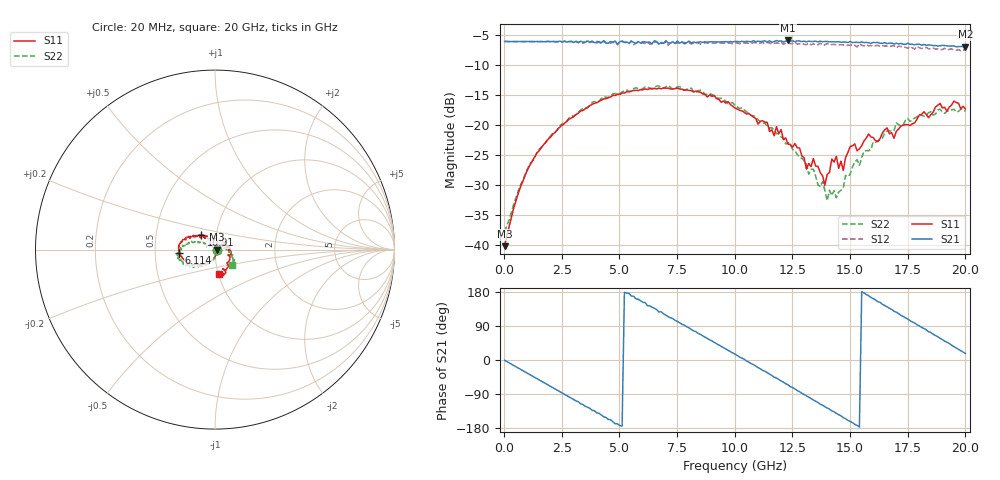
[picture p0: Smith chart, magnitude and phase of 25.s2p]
!Agilent Technologies,N5230A,US43500223,A.07.50.48
!Agilent N5230A: A.07.50.48
!Date: Wednesday, October 07, 2015 12:05:37
!Correction: S11(Full 2 Port(1,2))
!S21(Full 2 Port(1,2))
!S12(Full 2 Port(1,2))
!S22(Full 2 Port(1,2))
!S2P File: Measurements: S11, S21, S12, S22:
# Hz S  RI  R 50
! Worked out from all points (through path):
!   201 points, 20 MHz to 20 GHz, reference 50 ohm
!   highest |S21| = -5.91 dB at 12.31 GHz (marker M1); lowest = -7.0 dB at 20 GHz (marker M2)
!   group delay of S21, straight-line fit = 97.4 ps
!   lowest |S11| = -40.2 dB at 20 MHz (marker M3), VSWR 1.02, Z = 51 - j0.0154 ohm
!   |S11| at or under -10 dB: start of sweep to end of sweep
!   |S22| runs from -37.8 to -13.4 dB; largest |S21 - S12| = 0.056
!   S11 on the Smith chart (normalised r, x): 20 MHz: 1.02, -0.00; 6.114 GHz: 0.67, -0.03; 10.91 GHz: 0.84, +0.14; 20 GHz: 1.01, -0.28
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2e7  0.00981 -0.000151  0.4972 -0.00634  0.4965 -0.00734  0.0129 -0.00112
6.194e8  0.00632 -0.0266  0.4615 -0.1812  0.4601 -0.1829  0.00927 -0.0271
1.4186e9  -0.0137 -0.0568  0.326 -0.3746  0.3217 -0.3763  -0.0116 -0.0579
2.6174e9  -0.0629 -0.0821  -0.00392 -0.4998  -0.0122 -0.5011  -0.0555 -0.0869
3.4166e9  -0.103 -0.0832  -0.2276 -0.4358  -0.2377 -0.4169  -0.0965 -0.0981
4.8152e9  -0.1662 -0.0593  -0.4906 -0.1042  -0.4909 -0.0935  -0.1603 -0.0881
6.1139e9  -0.1992 -0.0185  -0.4338 0.2341  -0.4117 0.2409  -0.2007 -0.0541
6.7133e9  -0.2029 0.00205  -0.283 0.3785  -0.2688 0.3855  -0.2064 -0.0479
8.012e9  -0.1899 0.0406  0.0446 0.4981  0.0683 0.4819  -0.2032 -0.00274
1.001e10  -0.1189 0.0715  0.4798 0.1304  0.474 0.1028  -0.1404 0.0372
1.09091e10  -0.0783 0.0822  0.474 -0.1365  0.4534 -0.1716  -0.1091 0.0412
1.23077e10  -0.0348 0.0601  0.2105 -0.4605  0.1657 -0.4573  -0.0613 0.0364
1.28072e10  -0.0247 0.0596  0.0567 -0.4978  0.0229 -0.4746  -0.0439 0.0316
1.31069e10  -0.0103 0.0418  -0.0405 -0.4905  -0.0639 -0.4631  -0.034 0.034
1.34066e10  -0.006 0.0524  -0.1335 -0.4782  -0.1559 -0.4483  -0.0287 0.0321
1.39061e10  0.01 0.0299  -0.2726 -0.415  -0.2741 -0.3758  -0.00695 0.0278
1.44056e10  0.0464 0.0293  -0.3824 -0.3094  -0.3828 -0.2655  0.00935 0.023
1.47053e10  0.0359 0.0219  -0.4341 -0.2293  -0.423 -0.1915  0.022 0.0205
1.5005e10  0.0622 0.0234  -0.4729 -0.1518  -0.444 -0.1209  0.0363 0.0141
1.67033e10  0.0781 -0.0328  -0.3485 0.3311  -0.3097 0.324  0.0883 -0.017
1.82018e10  0.0615 -0.1137  0.0568 0.4652  0.0768 0.434  0.0977 -0.0671
2e10  0.024 -0.134  0.4282 0.1328  0.4154 0.0863  0.0974 -0.0861
